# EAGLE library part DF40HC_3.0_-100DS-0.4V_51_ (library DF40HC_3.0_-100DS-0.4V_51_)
Mezzanine Connectors (Board to Board) SMD,P=0.4mm RoHS Source: Datasheet
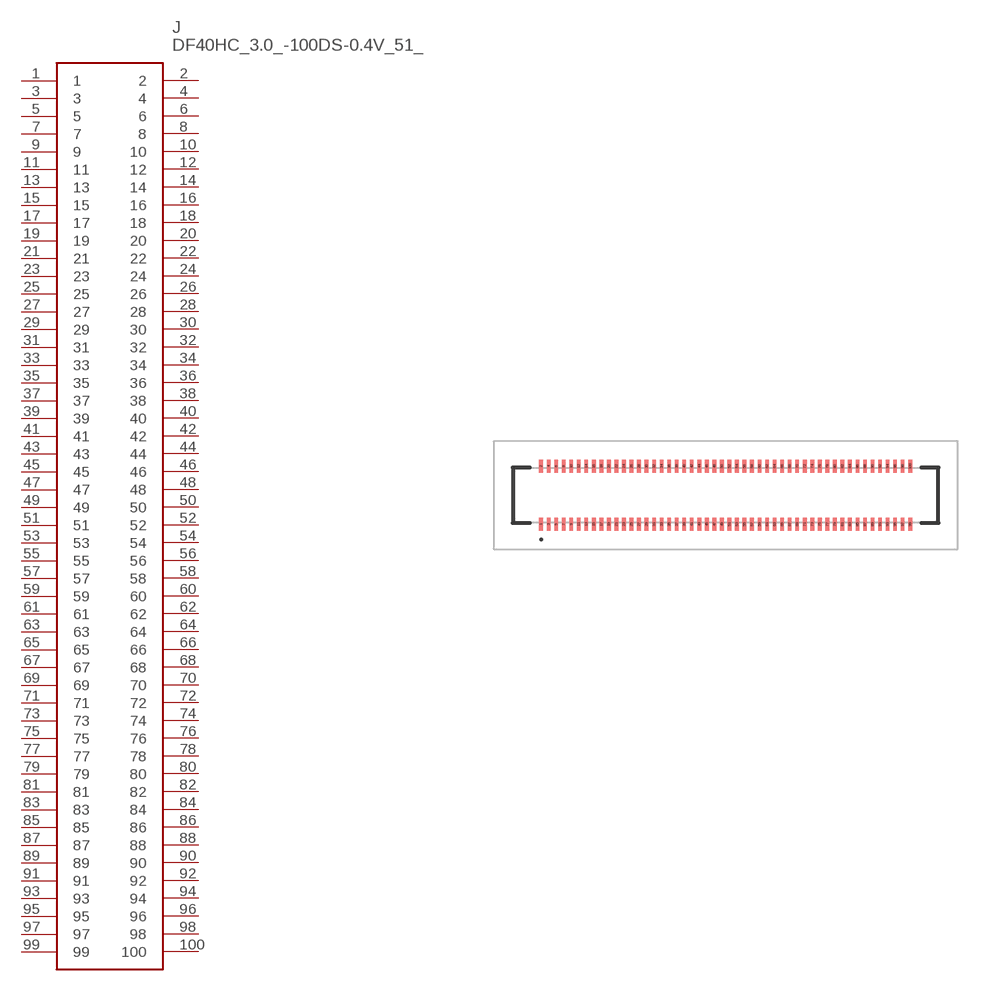
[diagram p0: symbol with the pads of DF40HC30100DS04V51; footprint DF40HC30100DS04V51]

Designator prefix J

## DF40HC_3.0_-100DS-0.4V_51_ (Description: Mezzanine Connectors (Board to Board) SMD,P=0.4mm RoHS; Height: 3.05mm; Manufacturer_Name: Hirose; Manufacturer_Part_Number: DF40HC(3.0)-100DS-0.4V(51))  [DF40HC30100DS04V51]
1  1
2  2
3  3
4  4
5  5
6  6
7  7
8  8
9  9
10  10
11  11
12  12
13  13
14  14
15  15
16  16
17  17
18  18
19  19
20  20
21  21
22  22
23  23
24  24
25  25
26  26
27  27
28  28
29  29
30  30
31  31
32  32
33  33
34  34
35  35
36  36
37  37
38  38
39  39
40  40
41  41
42  42
43  43
44  44
45  45
46  46
47  47
48  48
49  49
50  50
51  51
52  52
53  53
54  54
55  55
56  56
57  57
58  58
59  59
60  60
61  61
62  62
63  63
64  64
65  65
66  66
67  67
68  68
69  69
70  70
71  71
72  72
73  73
74  74
75  75
76  76
77  77
78  78
79  79
80  80
81  81
82  82
83  83
84  84
85  85
86  86
87  87
88  88
89  89
90  90
91  91
92  92
93  93
94  94
95  95
96  96
97  97
98  98
99  99
100  100

## Footprint DF40HC30100DS04V51 (pad centres in mm)
DF40HC(3.0)-100DS-0.4V(51)-1
smd 0.2 x 0.7: 1 -9.8,-1.54; 2 -9.8,1.54; 3 -9.4,-1.54; 4 -9.4,1.54; 5 -9,-1.54; 6 -9,1.54; 7 -8.6,-1.54; 8 -8.6,1.54; 9 -8.2,-1.54; 10 -8.2,1.54; 11 -7.8,-1.54; 12 -7.8,1.54; 13 -7.4,-1.54; 14 -7.4,1.54; 15 -7,-1.54; 16 -7,1.54; 17 -6.6,-1.54; 18 -6.6,1.54; 19 -6.2,-1.54; 20 -6.2,1.54; 21 -5.8,-1.54; 22 -5.8,1.54; 23 -5.4,-1.54; 24 -5.4,1.54; 25 -5,-1.54; 26 -5,1.54; 27 -4.6,-1.54; 28 -4.6,1.54; 29 -4.2,-1.54; 30 -4.2,1.54; 31 -3.8,-1.54; 32 -3.8,1.54; 33 -3.4,-1.54; 34 -3.4,1.54; 35 -3,-1.54; 36 -3,1.54; 37 -2.6,-1.54; 38 -2.6,1.54; 39 -2.2,-1.54; 40 -2.2,1.54; 41 -1.8,-1.54; 42 -1.8,1.54; 43 -1.4,-1.54; 44 -1.4,1.54; 45 -1,-1.54; 46 -1,1.54; 47 -0.6,-1.54; 48 -0.6,1.54; 49 -0.2,-1.54; 50 -0.2,1.54; 51 0.2,-1.54; 52 0.2,1.54; 53 0.6,-1.54; 54 0.6,1.54; 55 1,-1.54; 56 1,1.54; 57 1.4,-1.54; 58 1.4,1.54; 59 1.8,-1.54; 60 1.8,1.54; 61 2.2,-1.54; 62 2.2,1.54; 63 2.6,-1.54; 64 2.6,1.54; 65 3,-1.54; 66 3,1.54; 67 3.4,-1.54; 68 3.4,1.54; 69 3.8,-1.54; 70 3.8,1.54; 71 4.2,-1.54; 72 4.2,1.54; 73 4.6,-1.54; 74 4.6,1.54; 75 5,-1.54; 76 5,1.54; 77 5.4,-1.54; 78 5.4,1.54; 79 5.8,-1.54; 80 5.8,1.54; 81 6.2,-1.54; 82 6.2,1.54; 83 6.6,-1.54; 84 6.6,1.54; 85 7,-1.54; 86 7,1.54; 87 7.4,-1.54; 88 7.4,1.54; 89 7.8,-1.54; 90 7.8,1.54; 91 8.2,-1.54; 92 8.2,1.54; 93 8.6,-1.54; 94 8.6,1.54; 95 9,-1.54; 96 9,1.54; 97 9.4,-1.54; 98 9.4,1.54; 99 9.8,-1.54; 100 9.8,1.54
